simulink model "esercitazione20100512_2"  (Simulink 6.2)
settings: Solver=ode45  StartTime=0.0  StopTime=10  MaxStep=0.01  RelTol=1e-3
libraries: cstblocks x3

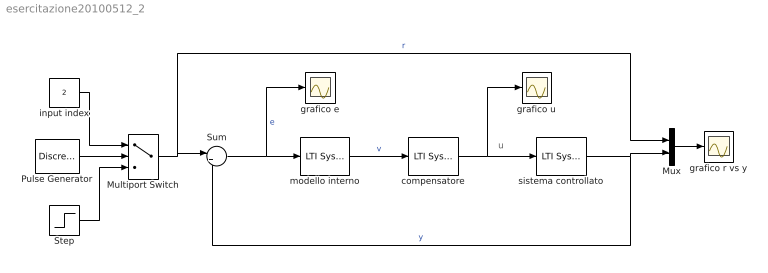
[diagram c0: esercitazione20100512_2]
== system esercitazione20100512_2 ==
  note: u
  Multiport Switch : MultiPortSwitch  Inputs=2
  Mux : Mux  Inputs=2
  Pulse Generator : DiscretePulseGenerator  PulseType=Time based  Period=10  PulseWidth=50
  Step : Step  Time=0  SampleTime=0
  Sum : Sum  Inputs=|+-
  compensatore : cstblocks/LTI System  sys=C  IC=0
  grafico e : Scope
  grafico r vs y : Scope
  grafico u : Scope
  input index : Constant  Value=2
  modello interno : cstblocks/LTI System  sys=M  IC=0
  sistema controllato : cstblocks/LTI System  sys=P  IC=0
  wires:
  modello interno/1 -> compensatore/1  "v"
  Multiport Switch/1 -> Sum/1, Mux/1  "r"
  compensatore/1 -> grafico u/1, sistema controllato/1
  sistema controllato/1 -> Sum/2, Mux/2  "y"
  Sum/1 -> grafico e/1, modello interno/1  "e"
  Pulse Generator/1 -> Multiport Switch/2
  Step/1 -> Multiport Switch/3
  input index/1 -> Multiport Switch/1
  Mux/1 -> grafico r vs y/1
